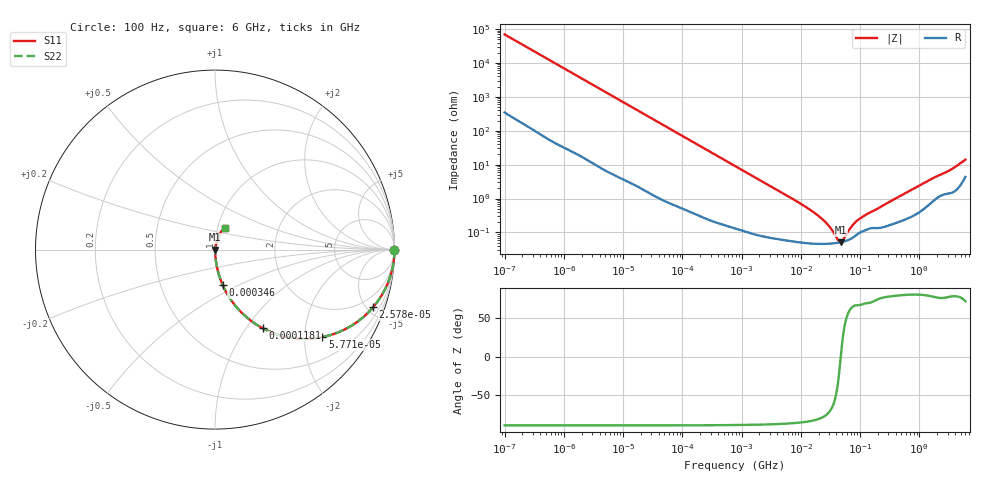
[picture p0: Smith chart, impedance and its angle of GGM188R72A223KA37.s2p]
!Murata Part Number: GGM188R72A223KA37
!These Parameters are Measured in Series Mode Connection
!Data Generated on Mar 13, 2026
!  o--ll--o
!Port1  Port2
!  o------o
!Operation Temp=25[degC], DC Bias Voltage=0[V]
!Freq. Start=100[Hz] Stop=6[GHz] 401[Steps]
# Hz S RI R 50
!Freq.(Hz) S11(Real) S11(Imag) S21(Real) S21(Imag) S12(Real) S12(Imag) S22(Real) S22(Imag)
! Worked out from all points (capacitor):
!   401 points, 100 Hz to 6 GHz, reference 50 ohm
!   read as one part in series: C = 23 nF near 109 Hz
!   lowest |Z| = 51.5 mohm at 47.65 MHz (marker M1)
!   series resonance near 47.33 MHz, so ESL is about 490 pH
!   S11 on the Smith chart (normalised r, x): 100 Hz: open; 25.78 kHz: 1.03, -5.46; 57.71 kHz: 1.02, -2.44; 118.1 kHz: 1.01, -1.20; 346 kHz: 1.00, -0.41; 6 GHz: 1.09, +0.27
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100  1 -0.00145  9.3e-06 0.00145  9.3e-06 0.00145  1 -0.00145
2008  0.999 -0.0288  0.000969 0.0288  0.000969 0.0288  0.999 -0.0288
8416  0.9852 -0.1183  0.0148 0.1183  0.0148 0.1183  0.9852 -0.1183
25777  0.8802 -0.3219  0.1198 0.3219  0.1198 0.3219  0.8802 -0.3219
40335  0.7518 -0.4291  0.2482 0.4291  0.2482 0.4291  0.7518 -0.4291
57709  0.5982 -0.4872  0.4018 0.4872  0.4018 0.4872  0.5982 -0.4872
118133  0.2653 -0.4378  0.7347 0.4378  0.7347 0.4378  0.2653 -0.4378
193316  0.1205 -0.3214  0.8795 0.3214  0.8795 0.3214  0.1205 -0.3214
345986  0.0422 -0.1962  0.9578 0.1962  0.9578 0.1962  0.0422 -0.1962
774597  0.00969 -0.0911  0.9903 0.0911  0.9903 0.0911  0.00969 -0.0911
1.555665e7  0.000485 -0.00419  0.9995 0.00419  0.9995 0.00419  0.000485 -0.00419
2.662322e7  0.000463 -0.00188  0.9995 0.00188  0.9995 0.00188  0.000463 -0.00188
3.330331e7  0.000472 -0.00111  0.9995 0.00111  0.9995 0.00111  0.000472 -0.00111
4.165952e7  0.000493 -0.000396  0.9995 0.000396  0.9995 0.000396  0.000493 -0.000396
4.764863e7  0.000515 2.14e-05  0.9995 -2.14e-05  0.9995 -2.14e-05  0.000515 2.14e-05
5.211241e7  0.000534 0.0003  0.9995 -0.0003  0.9995 -0.0003  0.000534 0.0003
7.129496e7  0.000661 0.00131  0.9993 -0.00131  0.9993 -0.00131  0.000661 0.00131
8.918374e7  0.000876 0.00205  0.9991 -0.00205  0.9991 -0.00205  0.000876 0.00205
3.124326e8  0.00168 0.00778  0.9983 -0.00778  0.9983 -0.00778  0.00168 0.00778
1.497423e9  0.00796 0.0345  0.992 -0.0345  0.992 -0.0345  0.00796 0.0345
3.205649e9  0.018 0.0634  0.982 -0.0634  0.982 -0.0634  0.018 0.0634
6e9  0.0571 0.1209  0.9429 -0.1209  0.9429 -0.1209  0.0571 0.1209
